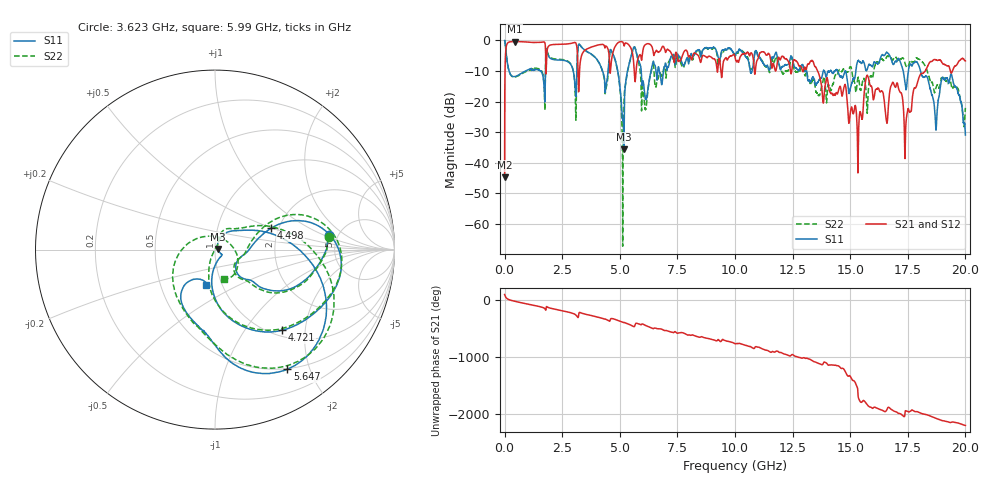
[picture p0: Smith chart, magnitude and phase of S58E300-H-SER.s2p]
!{S58E300}
!Johanson Technology Inc.
!www.johansontechnology.com
!Test Board Conditions:
!Substrate Type  RO4350B
!Substrate Thickness  60 mil
!Substrate Dk  3.66
!TL Type: GCPW
!TL Trace Width  115 mil
!TL Gap  52 mil
!Electrode orientation  Horizontal
!DUT TOPOLOGY	SERIES
!Mounting Pad LxW  55x428 mil
! Created Wed Apr 14 11:40:39 2021
# mhz S ma R 50
! 2 Port Network Data from SP1.SP block
! freq  magS11  angS11  magS21  angS21  magS12  angS12  magS22  angS22
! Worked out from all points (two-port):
!   20001 points, 300 kHz to 20 GHz, reference 50 ohm
!   highest |S21| = -0.34 dB at 438.3 MHz (marker M1); lowest = -44.7 dB at 300 kHz (marker M2)
!   |S21| within 3 dB of the highest: 49.94 MHz to 1.777 GHz (1.727 GHz wide, 189 % of centre); 1.845 GHz to 3.152 GHz (1.307 GHz wide, 52.3 % of centre)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
!   lowest |S11| = -35.6 dB at 5.178 GHz (marker M3), VSWR 1.03, Z = 51.7 + j0.355 ohm
!   |S11| at or under -10 dB: 13.11 GHz to 13.83 GHz (723.9 MHz wide, 5.37 % of centre); 14.45 GHz to 15.25 GHz (794.2 MHz wide, 5.35 % of centre); 18.05 GHz to end of sweep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
!   |S22| runs from -67.2 to 0.0 dB; largest |S21 - S12| = 0.0063
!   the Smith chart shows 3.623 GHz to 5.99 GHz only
!   S11 on the Smith chart (normalised r, x): 3.623 GHz: 4.23, +1.14; 4.498 GHz: 1.82, +0.49; 4.721 GHz: 1.11, -1.51; 5.647 GHz: 0.49, -1.66; 5.99 GHz: 0.84, -0.35
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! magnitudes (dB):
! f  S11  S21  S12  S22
! 300 kHz  0.0  -44.7  -44.9  0.0
! 114.3 MHz  -7.1  -1.0  -1.0  -7.1
! 438.3 MHz  -11.8  -0.3  -0.4  -12.0
! 3.043 GHz  -13.4  -0.7  -0.7  -14.1
! 3.334 GHz  -2.1  -5.1  -5.1  -2.1
! 3.623 GHz  -3.9  -2.6  -2.6  -3.9
! 4.498 GHz  -9.5  -3.0  -3.1  -10.6
! 4.721 GHz  -4.7  -3.5  -3.5  -4.8
! 5.178 GHz  -35.6  -1.6  -1.6  -21.6
! 5.647 GHz  -2.2  -12.5  -12.5  -2.1
! 5.99 GHz  -13.8  -4.0  -4.0  -15.3
! 6.667 GHz  -8.7  -3.9  -3.9  -12.3
! 10 GHz  -5.1  -5.3  -5.3  -5.1
! 13.33 GHz  -12.5  -6.6  -6.6  -13.5
! 15.36 GHz  -6.6  -30.1  -30.2  -12.2
! 15.74 GHz  -9.5  -11.4  -11.4  -23.8
! 16.67 GHz  -4.4  -20.5  -20.6  -5.3
! 17.42 GHz  -16.0  -27.0  -27.3  -8.4
! 17.91 GHz  -7.1  -14.1  -14.1  -5.8
! 18.71 GHz  -28.2  -6.3  -6.3  -15.8
! 19.41 GHz  -11.4  -10.5  -10.5  -15.4
! 20 GHz  -30.9  -6.7  -6.7  -22.0
